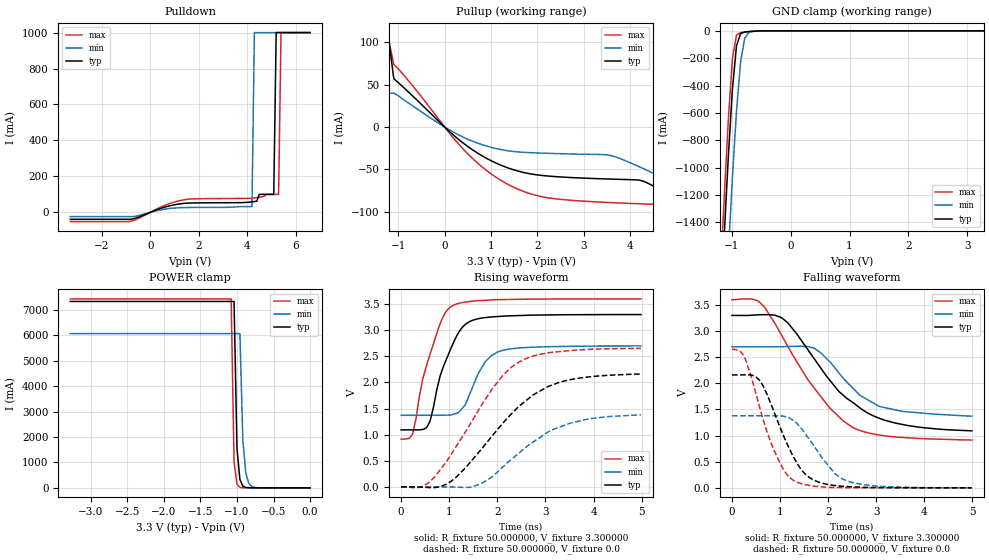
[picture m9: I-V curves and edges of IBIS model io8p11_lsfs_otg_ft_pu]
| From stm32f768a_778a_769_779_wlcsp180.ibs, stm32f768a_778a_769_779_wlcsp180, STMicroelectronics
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|   Model io8p11_lsfs_otg_ft_pu
[Model]  io8p11_lsfs_otg_ft_pu
Model_type I/O
Polarity   Non-Inverting
Enable   Active-Low
Vinl =   0.990000V
Vinh =   2.310000V
Vmeas =  1.650000V
Cref =   30.000000pF
Rref =   100.000000M
Vref =   0.0V
C_comp   8.196500pF   7.968500pF   8.492600pF
[Temperature Range]   25.000000   0.125000k   -40.000000
[Pullup Reference]   3.300000V   2.700000V   3.600000V
[Pulldown Reference]   0.0V   0.0V   0.0V
[POWER Clamp Reference]   3.300000V   2.700000V   3.600000V
[GND Clamp Reference]   0.0V   0.0V   0.0V
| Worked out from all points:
|   slope of the pulldown table from 0 to 0.495 V, typ, clamps not added: 20.1 ohm
|   slope of the pullup table from 0 to 0.495 V, typ, clamps not added: 21.8 ohm
|   GND clamp passes 1 mA (typ) near -0.52 V on its own axis
|   POWER clamp passes 1 mA (typ) near -0.80 V on its own axis
|   rising waveform, R_fixture 50.000000, V_fixture 3.300000: 20-80 % time 464ps typ, 428ps min, 454ps max; typ from 1.09 V to 3.3 V
|   rising waveform, R_fixture 50.000000, V_fixture 0.0: 20-80 % time 1.3ns typ, 1.18ns min, 1.13ns max; typ from 0.001 V to 2.16 V
|   falling waveform, R_fixture 50.000000, V_fixture 3.300000: 20-80 % time 1.24ns typ, 903ps min, 1.18ns max; typ from 3.3 V to 1.09 V
|   falling waveform, R_fixture 50.000000, V_fixture 0.0: 20-80 % time 624ps typ, 666ps min, 570ps max; typ from 2.16 V to 0.001 V
[Pulldown]
|Voltage   I(typ)   I(min)   I(max)
-3.3V     -38.65mA   -23.43mA   -51.3mA
-900mV    -38.65mA   -23.43mA   -51.3mA
1.4V      49.88mA    26.66mA    69.84mA
4.2V      58.43mA    32mA       78.86mA
4.3V      60.2mA     1A         80.13mA
4.4V      62mA       1A         81.72mA
4.5V      100mA      1A         83.79mA
5.1V      100mA      1A         100mA
5.2V      1A         1A         100mA
5.3V      1A         1A         100mA
5.4V      1A         1A         1A
6.6V      1A         1A         1A
[Pullup]
|Voltage   I(typ)   I(min)   I(max)
-3.3V     1A         1A         100mA
-1.9V     1A         1A         100mA
-1.8V     100mA      1A         100mA
-1.6V     100mA      1A         100mA
-1.5V     100mA      40mA       100mA
-1.2V     100mA      40mA       100mA
-1.1V     57mA       40mA       74mA
500mV     -22.94mA   -14.36mA   -31.63mA
1.6V      -52.16mA   -29.4mA    -73.72mA
4.2V      -62.55mA   -46.7mA    -90.52mA
5.5V      -103mA     -65mA      -126.2mA
6.6V      -103mA     -65mA      -139mA
[GND_clamp]
|Voltage   I(typ)   I(min)   I(max)
-3.3V     -9.479A    -9.465A    -9.974A
-1.2V     -2.125A    -2.854A    -1.857A
-1.13V    -1.511A    -2.236A    -1.236A
-1.06V    -933.3mA   -1.641A    -660.9mA
-990mV    -433.3mA   -1.082A    -206.9mA
-920mV    -110.3mA   -591mA     -31.45mA
-850mV    -19.78mA   -226.7mA   -13.65mA
-780mV    -8.311mA   -53.93mA   -9.506mA
-710mV    -5.285mA   -11.94mA   -6.262mA
-640mV    -3.232mA   -4.282mA   -3.577mA
3.28V     0A         0A         0A
[POWER_clamp]
|Voltage   I(typ)   I(min)   I(max)
-3.28V    7.329A     6.064A     7.43A
-1.08V    7.329A     6.064A     7.43A
-1.04V    7.329A     6.064A     1.015A
-1V       1.545A     6.064A     138.8mA
-960mV    325.8mA    6.064A     19.13mA
-920mV    68.77mA    1.89A      2.772mA
-880mV    14.59mA    589.1mA    520.3uA
-840mV    3.154mA    183.6mA    196.4uA
-800mV    734.4uA    57.27mA    136.6uA
-720mV    96.98uA    5.605mA    116.8uA
0V        0A         0A         0A
[Ramp]
| variable   typ   min   max
dV/dt_r  1.26819/1.27423n   0.78838/1.11234n   1.58109/1.12268n
dV/dt_f  1.28358/1.20525n   0.74820/0.85203n   1.59009/1.16429n
R_load = 50.000000
[Rising Waveform]
R_fixture= 50.000000
V_fixture= 3.300000
V_fixture_min= 2.700000
V_fixture_max= 3.600000
|time   V(typ)   V(min)   V(max)
0s        1.092V     1.372V     916mV
240.2ps   1.092V     1.372V     1.023V
530.5ps   1.139V     1.372V     2.333V
600.6ps   1.26V      1.372V     2.54V
840.8ps   2.207V     1.372V     3.193V
1.051ns   2.685V     1.38V      3.46V
1.381ns   3.143V     1.68V      3.545V
1.742ns   3.241V     2.388V     3.572V
2.002ns   3.262V     2.582V     3.585V
4.985ns   3.3V       2.7V       3.6V
[Rising Waveform]
R_fixture= 50.000000
V_fixture= 0.0
V_fixture_min= 0.0
V_fixture_max= 0.0
|time   V(typ)   V(min)   V(max)
0s        1.091mV    1.04mV     622.9uV
500.5ps   -6.29mV    1.066mV    38.15mV
700.7ps   -11.25mV   1.067mV    194.7mV
1.031ns   104mV      -881.1uV   611.4mV
1.652ns   705.2mV    56.75mV    1.534V
2.102ns   1.206V     371.9mV    2.12V
2.432ns   1.53V      635.9mV    2.379V
3.053ns   1.922V     1.05V      2.566V
3.504ns   2.051V     1.218V     2.61V
4.985ns   2.161V     1.38V      2.652V
[Falling Waveform]
R_fixture= 50.000000
V_fixture= 3.300000
V_fixture_min= 2.700000
V_fixture_max= 3.600000
|time   V(typ)   V(min)   V(max)
0s        3.3V       2.7V       3.6V
540.5ps   3.311V     2.7V       3.58V
680.7ps   3.315V     2.7V       3.455V
1.031ns   3.256V     2.701V     2.922V
1.712ns   2.468V     2.672V     1.909V
2.222ns   1.845V     2.202V     1.363V
2.523ns   1.627V     1.901V     1.149V
3.063ns   1.333V     1.559V     1.011V
3.934ns   1.156V     1.433V     942.7mV
4.985ns   1.092V     1.372V     916mV
[Falling Waveform]
R_fixture= 50.000000
V_fixture= 0.0
V_fixture_min= 0.0
V_fixture_max= 0.0
|time   V(typ)   V(min)   V(max)
0s        2.161V     1.38V      2.652V
240.2ps   2.163V     1.38V      2.54V
580.6ps   2.051V     1.38V      1.527V
930.9ps   1.319V     1.38V      606.9mV
1.111ns   914.4mV    1.362V     294.7mV
1.281ns   586.6mV    1.287V     143mV
1.672ns   163.6mV    845mV      37mV
2.142ns   44.93mV    270.4mV    7.288mV
2.372ns   25.31mV    141.1mV    4.463mV
4.985ns   1.091mV    1.04mV     622.9uV
